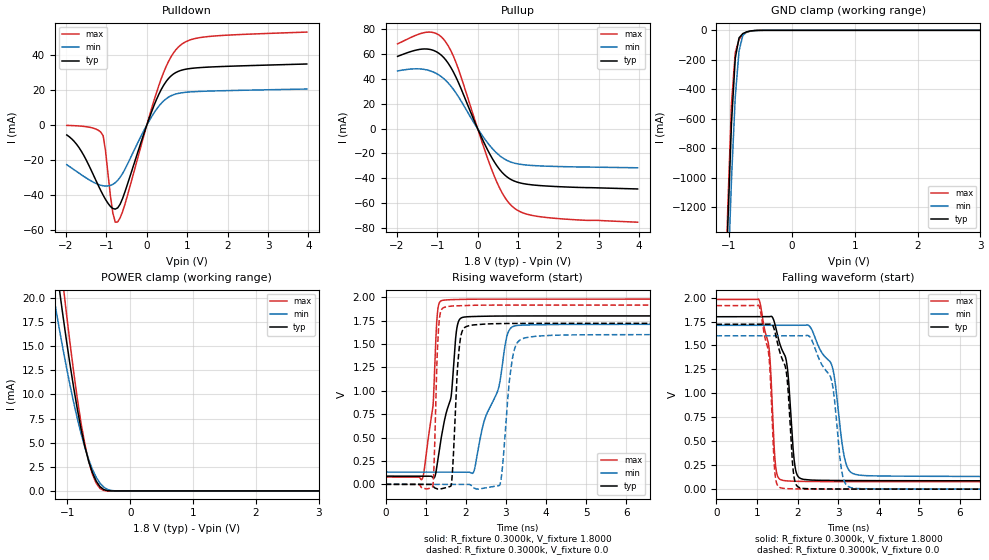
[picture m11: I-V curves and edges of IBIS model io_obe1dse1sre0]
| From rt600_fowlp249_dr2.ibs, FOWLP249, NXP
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[Model] io_obe1dse1sre0
|   Model io_obe1dse1sre0
| Library cells for typ/min/max conditions are connected as defined below:
|  pad - External Pad
|  ipp_do - Core Input
|  ipp_obe - Output Buffer Enable
|  REFH3V3 - vdd1v8
|  REFL3V3 - REFL3V3
|  gnde - gnde
|  ipp_dse - vdd
|  ipp_ina235_3v - NC
|  ipp_ina40_3v - NC
|  ipp_ina_mux - NC
|  ipp_ind - NC
|  ipp_ind_1p8v - NC
|  ipp_ind_3v - NC
|  vdd - vdd
|  vdd1v8 - vdd1v8
|  vdda - vdde3v3
|  vdde3v3 - vdde3v3
| All other pins connected to ground
Model_type I/O
Polarity   Non-Inverting
Enable   Active-High
Vinl =   0.5400V
Vinh =   1.2600V
Vmeas =  0.9000V
Cref =   25.0000pF
Rref =   0.5000k
Vref =   0.0V
C_comp   2.2457pF   2.1702pF   2.3895pF
[Temperature Range]   25.0000   0.1250k   -40.0000
[Voltage Range]   1.8000V   1.7100V   1.9800V
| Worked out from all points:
|   slope of the pulldown table from 0 to 0.27 V, typ, clamps not added: 16.6 ohm
|   slope of the pullup table from 0 to 0.27 V, typ, clamps not added: 14.6 ohm
|   GND clamp passes 1 mA (typ) near -0.57 V on its own axis
|   POWER clamp passes 1 mA (typ) near -0.54 V on its own axis
|   rising waveform, R_fixture 0.3000k, V_fixture 1.8000: 20-80 % time 364ps typ, 609ps min, 205ps max; typ from 0.087 V to 1.8 V
|   rising waveform, R_fixture 0.3000k, V_fixture 0.0: 20-80 % time 124ps typ, 198ps min, 81.7ps max; typ from 0 V to 1.72 V
|   falling waveform, R_fixture 0.3000k, V_fixture 1.8000: 20-80 % time 274ps typ, 456ps min, 191ps max; typ from 1.8 V to 0.087 V
|   falling waveform, R_fixture 0.3000k, V_fixture 0.0: 20-80 % time 258ps typ, 419ps min, 181ps max; typ from 1.72 V to 0 V
[Pulldown]
|Voltage   I(typ)   I(min)   I(max)
-1.98V    -5.65mA    -22.75mA   -160uA
-1.62V    -14.97mA   -28.49mA   -590uA
-1.08V    -40.24mA   -34.85mA   -6.067mA
-840mV    -47.89mA   -34.01mA   -50.49mA
-780mV    -48.24mA   -33.06mA   -55.75mA
-720mV    -47.53mA   -31.71mA   -55.6mA
-540mV    -38.27mA   -25.32mA   -45.39mA
240mV     14.7mA     9.107mA    18.7mA
540mV     26.85mA    16.1mA     36.66mA
780mV     30.9mA     18.23mA    44.81mA
1.44V     33.22mA    19.47mA    50.67mA
3.96V     35.11mA    20.73mA    53.44mA
[Pullup]
|Voltage   I(typ)   I(min)   I(max)
-1.98V    58.06mA    46.32mA    68.12mA
-1.2V     63.76mA    46.68mA    77.56mA
-960mV    60.59mA    43.12mA    75.31mA
-780mV    54.85mA    38.42mA    69.22mA
-480mV    37.43mA    25.91mA    48.3mA
60mV      -4.38mA    -2.967mA   -5.982mA
420mV     -27.07mA   -17.98mA   -38.74mA
660mV     -36.95mA   -24.37mA   -54.58mA
900mV     -42.07mA   -27.66mA   -63.71mA
1.2V      -44.59mA   -29.25mA   -68.57mA
1.68V     -46.09mA   -30.15mA   -71.35mA
3.96V     -48.5mA    -31.49mA   -75.21mA
[GND_clamp]
|Voltage   I(typ)   I(min)   I(max)
-1.98V    -17.57A    -17.55A    -18.13A
-1.08V    -2.185A    -2.567A    -2.121A
-1.02V    -1.339A    -1.74A     -1.223A
-960mV    -630.1mA   -1.012A    -499.4mA
-900mV    -189.5mA   -452.2mA   -152mA
-840mV    -51.34mA   -139.9mA   -62.86mA
-780mV    -22.28mA   -35.54mA   -26.58mA
-720mV    -10.62mA   -11.15mA   -13.18mA
-600mV    -1.527mA   -2.152mA   -2.249mA
-480mV    -85.63uA   -243.9uA   -63.17uA
3.96V     0A         0A         0A
[POWER_clamp]
|Voltage   I(typ)   I(min)   I(max)
-1.98V    66.18mA    51.42mA    77.85mA
-1.26V    27.66mA    21.8mA     33.09mA
-1.2V     24.56mA    19.48mA    29.34mA
-1.14V    21.54mA    17.24mA    25.67mA
-1.08V    18.63mA    15.07mA    22.11mA
-1.02V    15.84mA    13mA       18.69mA
-840mV    8.434mA    7.464mA    9.5mA
-720mV    4.556mA    4.476mA    4.785mA
-600mV    1.876mA    2.218mA    1.703mA
-540mV    1.008mA    1.402mA    786.9uA
-420mV    135uA      383.7uA    43.39uA
3.96V     0A         0A         0A
[Ramp]
| variable   typ   min   max
dV/dt_r  0.8235/0.2174n   0.6782/0.4113n   0.9804/0.1176n
dV/dt_f  0.7767/0.3509n   0.5489/0.6070n   0.9301/0.2311n
R_load = 50.0000
[Rising Waveform]
R_fixture= 0.3000k
V_fixture= 1.8000
V_fixture_min= 1.7100
V_fixture_max= 1.9800
|time   V(typ)   V(min)   V(max)
0s        87.44mV    130.7mV    78.02mV
917.7ps   87.44mV    130.7mV    61.1mV
1.221ns   74.42mV    130.7mV    1.209V
1.332ns   347.8mV    130.7mV    1.931V
1.635ns   941mV      130.7mV    1.974V
1.797ns   1.711V     130.7mV    1.976V
2.229ns   1.794V     182.9mV    1.979V
3.073ns   1.799V     1.641V     1.98V
4.386ns   1.8V       1.708V     1.98V
500ns     1.8V       1.71V      1.98V
[Rising Waveform]
R_fixture= 0.3000k
V_fixture= 0.0
V_fixture_min= 0.0
V_fixture_max= 0.0
|time   V(typ)   V(min)   V(max)
0s        22.64nV    701nV      38.04nV
1.174ns   -13.57mV   685.8nV    -25.35mV
1.335ns   -51.4mV    619.3nV    1.741V
1.629ns   -17.51mV   214.7nV    1.904V
1.872ns   1.575V     423.4nV    1.91V
2.345ns   1.71V      -49.16mV   1.915V
2.856ns   1.718V     3.015mV    1.915V
3.292ns   1.72V      1.518V     1.916V
4.718ns   1.721V     1.597V     1.916V
500ns     1.721V     1.6V       1.916V
[Falling Waveform]
R_fixture= 0.3000k
V_fixture= 1.8000
V_fixture_min= 1.7100
V_fixture_max= 1.9800
|time   V(typ)   V(min)   V(max)
0s        1.8V       1.71V      1.98V
1.052ns   1.8V       1.71V      1.976V
1.383ns   1.793V     1.71V      809.5mV
1.518ns   1.585V     1.71V      125.8mV
1.953ns   200.7mV    1.71V      82.21mV
2.268ns   96.57mV    1.711V     80.1mV
2.86ns    91.01mV    1.272V     78.76mV
3.254ns   89.95mV    206.5mV    78.39mV
4.415ns   88.33mV    136.1mV    78.08mV
500ns     87.44mV    130.7mV    78.02mV
[Falling Waveform]
R_fixture= 0.3000k
V_fixture= 0.0
V_fixture_min= 0.0
V_fixture_max= 0.0
|time   V(typ)   V(min)   V(max)
0s        1.721V     1.6V       1.916V
1.055ns   1.721V     1.6V       1.909V
1.386ns   1.712V     1.6V       590.2mV
1.723ns   1.225V     1.6V       5.872mV
1.926ns   97.93mV    1.6V       2.856mV
2.244ns   4.817mV    1.605V     1.295mV
2.836ns   1.573mV    1.14V      437.8uV
3.157ns   1.074mV    76.69mV    248.5uV
3.905ns   537.9uV    2.659mV    74.44uV
500ns     392.9nV    1.162uV    270.7nV
